TYPE E_HomeMode :
(
	ABSOLUTESWITCH 	:= 0,	(* 寻原点或寻原点辅助限位方式*)
	LIMITSWITCH 	:= 1, 	(* 寻限位开关方式*)
	DIRECTHOME		:= 2,	(* 直接回零 - *)
	ZPULSEHOME		:= 3,	(* 直接Z脉冲回零*)
	SETPOSITION		:= 4,	(* 直接设定位置*)
	BLOCKHOME		:= 5,	(* 堵转回零*)
	COEDRIVERHOME	:= 6	(* COE驱动器回零 *)
);
END_TYPE
